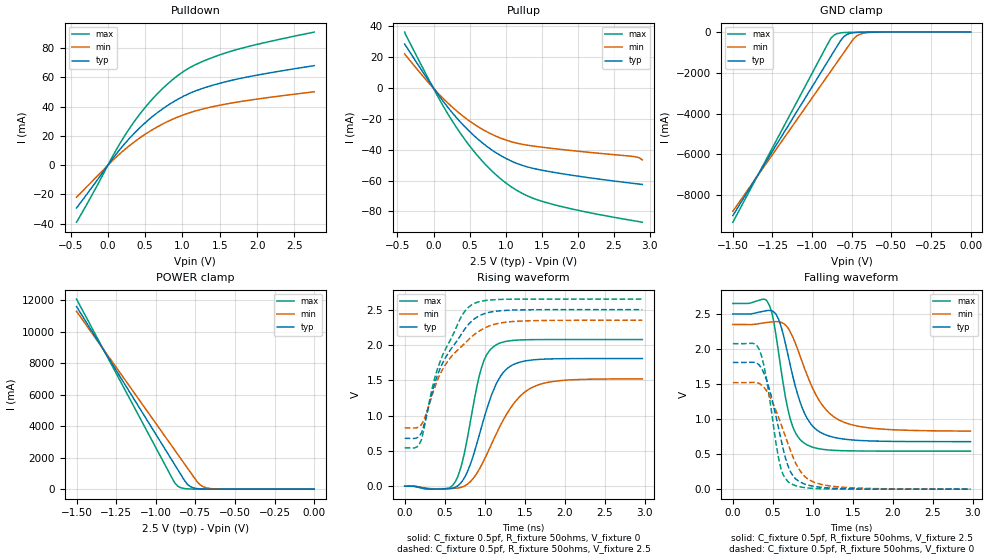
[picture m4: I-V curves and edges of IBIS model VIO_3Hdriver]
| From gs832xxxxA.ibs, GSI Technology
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|  signals   DQA1-DQA9, DQB1-DQB9, DQC1-DQC9, DQD1-DQD9
[Model]   VIO_3Hdriver
Model_type   I/O
Polarity   Non-Inverting
Vinl  =   0.80v
Vinh  =   2.00v
Vmeas =   1.25v
Cref  =   0pF
Rref  =   50
Vref  =   1.25v
|  variable   typ   min   max
C_comp   3.0pF   2.5pF   3.5pF
|  variable   typ   min   max
[Temperature Range]   50   0   100
|  variable   typ   min   max
[Voltage Range]   2.5   2.35   2.65
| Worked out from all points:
|   slope of the pulldown table from 0 to 0.375 V, typ, clamps not added: 16.4 ohm
|   slope of the pullup table from 0 to 0.375 V, typ, clamps not added: 16.9 ohm
|   GND clamp passes 1 mA (typ) near -0.58 V on its own axis
|   POWER clamp passes 1 mA (typ) near -0.61 V on its own axis
|   rising waveform, C_fixture 0.5pf, R_fixture 50ohms, V_fixture 0: 20-80 % time 307ps typ, 433ps min, 221ps max; typ from 0 V to 1.81 V
|   rising waveform, C_fixture 0.5pf, R_fixture 50ohms, V_fixture 2.5: 20-80 % time 418ps typ, 471ps min, 370ps max; typ from 0.678 V to 2.5 V
|   falling waveform, C_fixture 0.5pf, R_fixture 50ohms, V_fixture 2.5: 20-80 % time 269ps typ, 373ps min, 193ps max; typ from 2.5 V to 0.678 V
|   falling waveform, C_fixture 0.5pf, R_fixture 50ohms, V_fixture 0: 20-80 % time 230ps typ, 312ps min, 171ps max; typ from 1.81 V to 0 V
[Pulldown]
| voltage   typ   min   max
-420mV    -29.22mA   -21.86mA   -38.93mA
-210mV    -14.85mA   -10.95mA   -20.09mA
105mV     7.203mA    5.232mA    9.895mA
315mV     19.76mA    14.4mA     27.02mA
455mV     26.89mA    19.63mA    36.69mA
595mV     33.13mA    24.2mA     45.12mA
735mV     38.55mA    28.17mA    52.45mA
910mV     44.27mA    32.34mA    60.19mA
1.19V     51.06mA    37.31mA    69.09mA
1.575V    56.97mA    41.74mA    76.69mA
1.96V     61.18mA    44.91mA    82.09mA
2.765V    68.04mA    50.21mA    90.98mA
[Pullup]
| voltage (VDDQ-Vout) typ   min   max
-400mV    28.37mA    22.19mA    36.15mA
25mV      -1.684mA   -1.543mA   -2.625mA
305mV     -18.57mA   -14.3mA    -24.69mA
445mV     -25.69mA   -19.59mA   -34.12mA
620mV     -33.38mA   -25.2mA    -44.44mA
795mV     -39.75mA   -29.74mA   -53.17mA
970mV     -44.85mA   -33.21mA   -60.37mA
1.25V     -50.46mA   -36.68mA   -68.78mA
1.53V     -53.53mA   -38.54mA   -73.8mA
2.055V    -57.5mA    -41.25mA   -79.77mA
2.755V    -61.75mA   -44.32mA   -85.86mA
2.895V    -62.54mA   -46.64mA   -86.96mA
[GND Clamp]
| voltage   typ   min   max
-1.5V     -9.007A    -8.796A    -9.334A
-900mV    -1.426A    -2.122A    -562.9mA
-880mV    -1.172A    -1.9A      -292.9mA
-860mV    -920.8mA   -1.678A    -142.5mA
-820mV    -415.8mA   -1.233A    -38.58mA
-800mV    -225.7mA   -1.011A    -23.51mA
-780mV    -116.6mA   -788.8mA   -16.2mA
-740mV    -28.49mA   -348.7mA   -9.876mA
-720mV    -19.99mA   -198.2mA   -8.142mA
-680mV    -4.537mA   -61.92mA   -5.539mA
-580mV    -1.002mA   -3.885mA   -1.438mA
0V        -532.9pA   -960.9pA   -479.8pA
[POWER Clamp]
| voltage (VDDQ-Vout) typ   min   max
-1.5V     11.62A     11.31A     12.09A
-900mV    1.877A     2.767A     762.9mA
-880mV    1.552A     2.482A     397.9mA
-860mV    1.228A     2.198A     182.9mA
-840mV    903.1mA    1.913A     83.23mA
-800mV    303.9mA    1.344A     19.13mA
-780mV    154.4mA    1.059A     10.41mA
-740mV    39.27mA    489.6mA    4.442mA
-720mV    20.11mA    274.2mA    3.362mA
-680mV    5.757mA    82.61mA    2.175mA
-580mV    536.8uA    4.105mA    644.2uA
0V        760.5pA    2.222nA    488.1pA
[Ramp]
| voltage   typ   min   max
dV/dt_r   1.53/137p   1.35/170p   1.77/112p
dV/dt_f   1.51/136p   1.31/167p   1.77/112p
R_load  =   50ohms
[Rising Waveform]
C_fixture =   0.5pf
R_fixture =   50ohms
V_fixture =   0
| Time   V(typ)   V(min)   V(max)
0s        5.712nV    13.22nV    3.887nV
510ps     -36.21mV   -33.7mV    -36.31mV
630ps     -15.86mV   -28.86mV   58.71mV
720ps     72.97mV    -10.31mV   341.5mV
780ps     196.4mV    25.53mV    661.7mV
960ps     838.4mV    298.6mV    1.678V
1.14ns    1.44V      731.7mV    2V
1.38ns    1.734V     1.196V     2.067V
1.68ns    1.796V     1.439V     2.076V
2.97ns    1.808V     1.52V      2.077V
[Rising Waveform]
C_fixture =   0.5pf
R_fixture =   50ohms
V_fixture =   2.5
V_fixture_min =   2.35
V_fixture_max =   2.65
| Time   V(typ)   V(min)   V(max)
0s        678mV      826.7mV    543.2mV
150ps     683mV      827.6mV    553.9mV
210ps     755.9mV    872.9mV    661.3mV
360ps     1.399V     1.349V     1.466V
450ps     1.687V     1.603V     1.788V
720ps     2.173V     1.99V      2.426V
840ps     2.34V      2.12V      2.57V
1.02ns    2.452V     2.252V     2.631V
1.29ns    2.491V     2.326V     2.648V
2.97ns    2.5V       2.35V      2.65V
[Falling Waveform]
C_fixture =   0.5pf
R_fixture =   50ohms
V_fixture =   2.5
V_fixture_min =   2.35
V_fixture_max =   2.65
| Time   V(typ)   V(min)   V(max)
0s        2.5V       2.35V      2.65V
450ps     2.551V     2.382V     2.639V
510ps     2.532V     2.389V     2.4V
570ps     2.429V     2.39V      1.96V
660ps     2.062V     2.34V      1.295V
720ps     1.754V     2.239V     991.9mV
900ps     1.073V     1.71V      650.8mV
1.11ns    801.9mV    1.212V     571mV
1.38ns    715.9mV    958.9mV    548.8mV
2.97ns    678.3mV    829mV      543.3mV
[Falling Waveform]
C_fixture =   0.5pf
R_fixture =   50ohms
V_fixture =   0
| Time   V(typ)   V(min)   V(max)
0s        1.808V     1.52V      2.077V
330ps     1.772V     1.509V     1.993V
390ps     1.649V     1.451V     1.755V
450ps     1.45V      1.346V     1.361V
540ps     1.033V     1.117V     648.4mV
600ps     718.7mV    932.9mV    293.8mV
720ps     248.5mV    551mV      82mV
870ps     85.15mV    216mV      27.3mV
1.11ns    26.13mV    66.95mV    5.338mV
2.97ns    10.37uV    274.4uV    233.3nV
